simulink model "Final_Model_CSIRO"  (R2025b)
settings: Solver=ode23tb  StartTime=0.0  StopTime=50  RelTol=1e-3
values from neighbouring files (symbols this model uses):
  C_4 = 0.1670*C_b    (= 1.00487241952e-06)    [VSM_CSIRO.m]    (also in VSM.m)
  C_6 = 0.2835*C_b    (= 1.70587623314e-06)    [VSM_CSIRO.m]    (also in VSM.m)
  C_8 = 0.2275*C_b    (= 1.36891302659e-06)    [VSM_CSIRO.m]    (also in VSM.m)
  C_dc = 0.008*(n)    (= 1.6)    [VSM_CSIRO.m]    (also in VSM.m)
  C_f = n*300*10^-6    (= 0.06)    [VSM_CSIRO.m]    (also in VSM.m)
  D_p = (1/(m_p*w_b))    (= 101321.183642)    [VSM_CSIRO.m]    (also in VSM.m)
  droop_percentage = 1    [VSM_CSIRO.m]    (also in VSM.m = 5)
  i_ll = -1.15*(S_b/Vdc_n)-i_loss_dc    [VSM_CSIRO.m]    (also in VSM.m)
  i_ul = 1.15*(S_b/Vdc_n)+i_loss_dc    [VSM_CSIRO.m]    (also in VSM.m)
  J = D_p*tau_f    (= 2026.42367285)    [VSM_CSIRO.m]    (also in VSM.m)
  k_dc = eta_1/(Vdc_n*m_p)    [VSM_CSIRO.m]    (also in VSM.m)
  K_p = (1/Vdc_n)    [VSM_CSIRO.m]    (also in VSM.m)
  K_r = 1/R_dc    [VSM_CSIRO.m]    (also in VSM.m)
  Kff_i = 1    [VSM_CSIRO.m]    (also in VSM.m)
  Kff_v = 1    [VSM_CSIRO.m]    (also in VSM.m)
  Ki_i = (1/n)*1.19    (= 0.00595)    [VSM_CSIRO.m]    (also in VSM.m)
  Ki_v = (n)*1.161022    (= 232.2044)    [VSM_CSIRO.m]    (also in VSM.m)
  ki_v_ac = 4*5.2500e-04    (= 0.0021)    [VSM_CSIRO.m]    (also in VSM.m)
  Kp_i = 0.738891    [VSM_CSIRO.m]    (also in VSM.m)
  Kp_v = 0.52    [VSM_CSIRO.m]    (also in VSM.m)
  kp_v_ac = 0.001    [VSM_CSIRO.m]    (also in VSM.m)
  L1_pu = 1*0.0186/m    (= 0.000186)    [VSM_CSIRO.m]    (also in VSM.m)
  L_45 = L_lines(2)    [VSM_CSIRO.m]    (also in VSM.m)
  L_56 = L_lines(3)    [VSM_CSIRO.m]    (also in VSM.m)
  L_67 = L_lines(5)    [VSM_CSIRO.m]    (also in VSM.m)
  L_78 = L_lines(6)    [VSM_CSIRO.m]    (also in VSM.m)
  L_89 = L_lines(8)    [VSM_CSIRO.m]    (also in VSM.m)
  L_94 = L_lines(9)    [VSM_CSIRO.m]    (also in VSM.m)
  L_f = (1/n)*200*10^-6    (= 1e-06)    [VSM_CSIRO.m]    (also in VSM.m)
  n = 200    [VSM_CSIRO.m]    (also in VSM.m)
  pl = S_b*ps    (= 75000000)    [VSM_CSIRO.m]    (also in VSM.m)
  ps = base/3    (= 0.75)    [VSM_CSIRO.m]    (also in VSM.m)
  R1_pu = 1*0.00734/m    (= 7.34e-05)    [VSM_CSIRO.m]    (also in VSM.m)
  R_45 = R_lines(2)    [VSM_CSIRO.m]    (also in VSM.m)
  R_56 = R_lines(3)    [VSM_CSIRO.m]    (also in VSM.m)
  R_67 = R_lines(5)    [VSM_CSIRO.m]    (also in VSM.m)
  R_78 = R_lines(6)    [VSM_CSIRO.m]    (also in VSM.m)
  R_89 = R_lines(8)    [VSM_CSIRO.m]    (also in VSM.m)
  R_94 = R_lines(9)    [VSM_CSIRO.m]    (also in VSM.m)
  R_dc = (Vdc_n/(0.05*(S_b)/Vdc_n))    [VSM_CSIRO.m]    (also in VSM.m)
  R_f = 0.001/n    (= 5e-06)    [VSM_CSIRO.m]    (also in VSM.m)
  S_b = 100*(10^6)    (= 100000000)    [VSM_CSIRO.m]    (also in VSM.m)
  S_bt = S_b    (= 100000000)    [VSM_CSIRO.m]    (also in VSM.m)
  T_en = T_load-0.5    (= 44.5)    [VSM_CSIRO.m]    (also in VSM.m = 24.5)
  t_l = 2    [VSM_CSIRO.m]
  tau_dc = 0.05    [VSM_CSIRO.m]    (also in VSM.m)
  tau_g = 5    [VSM_CSIRO.m]    (also in VSM.m)
  V1_rms = 1000    [VSM_CSIRO.m]    (also in VSM.m)
  V2_rms = 13800    [VSM_CSIRO.m]    (also in VSM.m)
  V_m = sqrt(2/3)*V1_rms    [VSM_CSIRO.m]    (also in VSM.m)
  Vdc_n = 3*V_m    [VSM_CSIRO.m]    (also in VSM.m)
  w_b = 2*pi*f_b    (= 314.159265359)    [VSM_CSIRO.m]    (also in VSM.m)
  w_f = 2*pi*5    (= 31.4159265359)    [VSM_CSIRO.m]    (also in VSM.m)
undefined symbols (not defined in the file or in its folder): D1, Delta, DiscIntNeverNeededParam, i_dc
libraries: spsSeriesRLCBranchLib x142, spsThreePhaseVIMeasurementLib x69, slpidlib x44, spsabctodq0Lib x44, spsVoltageMeasurementLib x28, spsGroundLib x23, spsThreePhaseBreakerLib x23, spsThreePhaseParallelRLCLoadLib x21, spsdq0toabcLib x16, spsUniversalBridgeLib x16, spsPowerPositiveSequenceLib x14, spsDCVoltageSourceLib x14
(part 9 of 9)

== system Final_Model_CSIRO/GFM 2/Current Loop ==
  i_s_ref_dq0 : Inport
  v_dq0 : Inport  Port=2
  i_s_dq0 : Inport  Port=3
  w : Inport  Port=4
  Demux : Demux  Outputs=2
  Demux1 : Demux  Outputs=2
  Demux2 : Demux  Outputs=2
  First-Order Filter2 : spsFirstOrderFilterLib/First-Order Filter  Commented=on  FilterType=Lowpass  Tc=25e-3  Ts=0  Initialize=on  Vac_Init=[0, 0, 50]  Vdc_Init=1  PlotResponse=off  FreqRange="[0,  200,  1]"
  First-Order Filter3 : spsFirstOrderFilterLib/First-Order Filter  Commented=on  FilterType=Lowpass  Tc=25e-3  Ts=0  Initialize=on  Vac_Init=[0, 0, 50]  Vdc_Init=0  PlotResponse=off  FreqRange="[0,  200,  1]"
  Gain Corrector : Gain  Gain=Kp_i
  Gain Corrector1 : Gain  Gain=Kp_i
  Integration Time : Gain  Gain=Ki_i / Kp_i
  Integration Time 1 : Gain  Gain=Ki_i / Kp_i
  Integration Time1 : Gain  Gain=1/n
  Integration Time2 : Gain  Gain=1/n
  Integrator : Integrator  InitialCondition=0.0001
  Integrator 1 : Integrator
  Mux : Mux  Inputs=3
  Product : Product  RndMeth=Zero
  Product1 : Product  RndMeth=Zero
  Selector1 : Selector  InputPortWidth=3  IndexOptions=Index vector (dialog)  Indices=[1 2]  OutputSizes=1
  Selector2 : Selector  InputPortWidth=3  IndexOptions=Index vector (dialog)  Indices=[1 2]  OutputSizes=1
  Selector3 : Selector  InputPortWidth=3  IndexOptions=Index vector (dialog)  Indices=[1 2]  OutputSizes=1
  Sum : Sum  Inputs=|+-
  Sum1 : Sum  Inputs=|++
  Sum2 : Sum  Inputs=|+-
  Sum3 : Sum  Inputs=|++
  Sum4 : Sum  Inputs=|++
  Sum5 : Sum  Inputs=++|
  Sum6 : Sum  Inputs=-+|
  Sum7 : Sum  Inputs=++|
  Vm_0* : Constant  Value=0
  Voltage Compensator 1 : Gain  Gain=Kff_v
  Voltage compensator : Gain  Gain=Kff_v
  w*Lf_pu : Gain  Gain=L_f
  v_s_ref_dq0 : Outport  VectorParamsAs1DForOutWhenUnconnected=off
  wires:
  Integration Time2/1 -> Sum4/2
  Integration Time1/1 -> Sum1/2
  Gain Corrector1/1 -> Sum5/2
  Product1/1 -> Sum5/1
  Demux2/1 -> Voltage compensator/1
  Demux1/1 -> Sum/2, Product1/2
  Integrator/1 -> Sum1/1
  Vm_0*/1 -> Mux/3
  Demux1/2 -> Sum6/1, Product/1
  Selector3/1 -> Demux2/1
  i_s_dq0/1 -> Selector2/1
  Selector2/1 -> Demux1/1
  Mux/1 -> v_s_ref_dq0/1
  w/1 -> w*Lf_pu/1
  Gain Corrector/1 -> Sum2/1
  Selector1/1 -> Demux/1
  Demux/2 -> Sum6/2
  Sum4/1 -> Gain Corrector1/1
  Sum2/1 -> Sum3/1
  Sum1/1 -> Gain Corrector/1
  Voltage compensator/1 -> Sum3/2
  Integrator 1/1 -> Sum4/1
  v_dq0/1 -> Selector3/1
  i_s_ref_dq0/1 -> Selector1/1
  w*Lf_pu/1 -> Product/2, Product1/1
  Product/1 -> Sum2/2
  Voltage Compensator 1/1 -> Sum7/1
  Demux2/2 -> Voltage Compensator 1/1
  Sum7/1 -> Mux/2  "Vm_q*"
  Sum3/1 -> Mux/1  "Vm_d*"
  Demux/1 -> Sum/1
  Sum6/1 -> Integration Time2/1, Integration Time 1/1
  Sum5/1 -> Sum7/2
  Integration Time/1 -> Integrator/1
  Integration Time 1/1 -> Integrator 1/1
  Sum/1 -> Integration Time1/1, Integration Time/1

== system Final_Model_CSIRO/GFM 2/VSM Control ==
  p_m : Inport
  p_set : Inport  Port=2
  v_m : Inport  Port=3
  V_abc : Inport  Port=4
  w_b : Inport  Port=5
  Demux : Demux  Outputs=3
  Gain17 : Gain  Gain=1/(w_b)
  Gain2 : Gain  Gain=1/(w_b)
  Gain5 : Gain  Gain=D_p
  Gain6 : Gain  Gain=1/J
  Integrator : Integrator
  Integrator2 : Integrator
  MATLAB Function1 : MATLAB Function  TreatAsAtomicUnit=on
  PID Controller : slpidlib/PID Controller  Controller=PID  Form=Parallel  TimeDomain=Continuous-time  UseExternalTs=off  SampleTime=-1  IntegratorMethod=Forward Euler  FilterMethod=Forward Euler  ControllerParametersSource=internal  P=kp_v_ac  I=ki_v_ac  UseKiTs=off  D=0  UseExternalDerivativeSource=off  N=100  UseFilter=on  TunerSelectOption=Transfer Function Based (PID Tuner App)  InitialConditionSource=internal  InitialConditionForIntegrator=0  InitialConditionForFilter=0  DifferentiatorICPrevScaledInput=0  ExternalReset=none  TrackingMode=off  Kt=1  LimitOutput=off  SatLimitsSource=internal  UpperSaturationLimit=inf  LowerSaturationLimit=-inf  LinearizeAsGain=on  AntiWindupMode=none  Kb=1  LimitIntegrator=off  UpperIntegratorSaturationLimit=inf  LowerIntegratorSaturationLimit=-inf  POutMin=[]  POutMax=[]  IOutMin=[]  IOutMax=[]  DOutMin=[]  DOutMax=[]  NOutMin=[]  NOutMax=[]  SumOutMin=[]  SumOutMax=[]  SaturationOutMin=[]  SaturationOutMax=[]  PParamMin=[]  PParamMax=[]  IParamMin=[]  IParamMax=[]  DParamMin=[]  DParamMax=[]  NParamMin=[]  NParamMax=[]  KbParamMin=[]  KbParamMax=[]  KtParamMin=[]  KtParamMax=[]  KbOutMin=[]  KbOutMax=[]  KtOutMin=[]  KtOutMax=[]  IntegratorOutMin=[]  IntegratorOutMax=[]  FilterOutMin=[]  FilterOutMax=[]  SumI1OutMin=[]  SumI1OutMax=[]  SumI2OutMin=[]  SumI2OutMax=[]  SumI3OutMin=[]  SumI3OutMax=[]  SumI4OutMin=[]  SumI4OutMax=[]  SumDOutMin=[]  SumDOutMax=[]  DifferentiatorOutMin=[]  DifferentiatorOutMax=[]  FilterDiffOutCoefMin=[]  FilterDiffOutCoefMax=[]  ReciprocalOutMin=[]  ReciprocalOutMax=[]  SumDenOutMin=[]  SumDenOutMax=[]  SumNumOutMin=[]  SumNumOutMax=[]  DivideOutMin=[]  DivideOutMax=[]  UdiffTsProdOutMin=[]  UdiffTsProdOutMax=[]  NTsProdOutMin=[]  NTsProdOutMax=[]  UintegralTsProdOutMin=[]  UintegralTsProdOutMax=[]  UngainTsProdOutMin=[]  UngainTsProdOutMax=[]  ClampingZeroOutDataTypeStr=Inherit: Inherit via back propagation  ClampingZeroOutMin=[]  ClampingZeroOutMax=[]  FilterDenConstantOutDataTypeStr=Inherit: Inherit via back propagation  FilterDenConstantOutMin=[]  FilterDenConstantOutMax=[]  PCopyOutDataTypeStr=Inherit: Inherit via back propagation  PCopyOutMin=[]  PCopyOutMax=[]  NCopyOutDataTypeStr=Inherit: Inherit via back propagation  NCopyOutMin=[]  NCopyOutMax=[]  IntegratorContinuousStateAttributes=''  IntegratorStateMustResolveToSignalObject=off  IntegratorRTWStateStorageClass=Auto  FilterContinuousStateAttributes=''  FilterStateMustResolveToSignalObject=off  FilterRTWStateStorageClass=Auto  ParallelPVariant=InternalParameters  IdealPVariant=Disabled  IVariant=InternalParameters  DVariant=InternalParameters  IntegratorVariant=Continuous  SatVariant=Disabled  AWVariant=Passthrough  PCopyVariant=Disabled  TRVariant=Disabled  FdbkBlocksVariant=Forward  IdealPFdbkVariant=Disabled  SatFdbkVariant=Disabled  DerivativeFilterVariant=ContFilter  NVariant=InternalParameters  NCopyVariant=Disabled  FilterICVariant=InternalICsFilter  IntegratorICVariant=InternalICs  ExternalResetVariant=Disabled  TRSumVariant=Passthrough  SumFdbkVariant=Disabled  SumVariant=Sum_PID  TsampFilterVariant=InternalTs  TsampNgainVariant=Passthrough  TsampIntegralVariant=Disabled_SignalSpec  ExternalSaturationOutDataTypeStr=Inherit: Same as second input  DerivativeSourceVariant=ErrorSignal  PreIntVariant=InternalPreInt
  Sum : Sum  Inputs=+|+|-
  Sum1 : Sum  Inputs=-+|
  Sum2 : Sum  Inputs=+|-
  Terminator : Terminator
  Terminator1 : Terminator
  Transfer Fcn1 : TransferFcn  Numerator=[w_f]  Denominator=[1 w_f]
  abc to dq1 : spsabctodq0Lib/abc to dq0  Alignment=90 degrees behind phase A axis
  abc to dq2 : spsabctodq0Lib/abc to dq0  Alignment=90 degrees behind phase A axis
  w_ref : Outport  VectorParamsAs1DForOutWhenUnconnected=off
  theta_ref : Outport  Port=2  VectorParamsAs1DForOutWhenUnconnected=off
  v_ref_dq0 : Outport  Port=3  VectorParamsAs1DForOutWhenUnconnected=off
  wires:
  v_m/1 -> Sum1/2
  Sum1/1 -> PID Controller/1
  abc to dq1/1 -> Demux/1
  V_abc/1 -> abc to dq1/1
  Demux/1 -> Sum1/1
  Demux/2 -> Terminator/1
  Demux/3 -> Terminator1/1
  w_b/1 -> Sum2/1
  Integrator/1 -> Integrator2/1, Sum2/2, w_ref/1, MATLAB Function1/3(w)
  Transfer Fcn1/1 -> Gain17/1
  Integrator2/1 -> abc to dq1/2, MATLAB Function1/2(theta), abc to dq2/2, theta_ref/1
  Sum2/1 -> Gain5/1
  Sum/1 -> Gain6/1
  Gain2/1 -> Sum/2
  Gain6/1 -> Integrator/1
  Gain17/1 -> Sum/3
  Gain5/1 -> Sum/1
  p_m/1 -> Transfer Fcn1/1
  p_set/1 -> Gain2/1
  PID Controller/1 -> MATLAB Function1/1(M_fi_f)
  MATLAB Function1/1(e) -> abc to dq2/1
  abc to dq2/1 -> v_ref_dq0/1

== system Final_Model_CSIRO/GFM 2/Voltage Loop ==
  v_ref_dq0 : Inport
  v_dq0 : Inport  Port=2
  i_dq0 : Inport  Port=3
  w : Inport  Port=4
  Current Compensator : Gain  Gain=Kff_i
  Current Compensator1 : Gain  Gain=Kff_i
  Damping (d) : Gain  Gain=Kp_v
  Damping (q) : Gain  Gain=Kp_v
  Demux : Demux  Outputs=2
  Demux1 : Demux  Outputs=2
  Demux2 : Demux  Outputs=2
  Eg_d * (wCf) : Product  RndMeth=Zero
  "Eg_q * (wCf) " : Product  RndMeth=Zero
  Filter capacitance : Gain  Gain=C_f
  Integration Time : Gain  Gain=Ki_v / Kp_v
  Integration Time1 : Gain  Gain=Ki_v / Kp_v
  Integration Time2 : Gain  Gain=n
  Integration Time3 : Gain  Gain=n
  Integrator : Integrator
  Integrator1 : Integrator
  Is_0* : Constant  Value=0
  Mux : Mux  Inputs=3
  Selector : Selector  InputPortWidth=3  IndexOptions=Index vector (dialog)  Indices=[1 2]  OutputSizes=1
  Selector1 : Selector  InputPortWidth=3  IndexOptions=Index vector (dialog)  Indices=[1 2]  OutputSizes=1
  Selector2 : Selector  InputPortWidth=3  IndexOptions=Index vector (dialog)  Indices=[1 2]  OutputSizes=1
  Sum : Sum  Inputs=|+-
  Sum1 : Sum  Inputs=|++
  Sum2 : Sum  Inputs=|+-
  Sum3 : Sum  Inputs=|++
  Sum4 : Sum  Inputs=|++
  Sum5 : Sum  Inputs=++|
  Sum6 : Sum  Inputs=-+|
  Sum7 : Sum  Inputs=++|
  i_s_ref_dq0 : Outport  VectorParamsAs1DForOutWhenUnconnected=off
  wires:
  Integration Time3/1 -> Sum4/2
  Integration Time2/1 -> Sum1/2
  Sum/1 -> Integration Time2/1, Integration Time/1
  Mux/1 -> i_s_ref_dq0/1
  Selector2/1 -> Demux2/1
  Selector1/1 -> Demux/1
  Selector/1 -> Demux1/1
  Damping (q)/1 -> Sum5/2  "Is_q\""
  v_dq0/1 -> Selector/1
  Sum3/1 -> Mux/1  "Is_d*"
  Sum4/1 -> Damping (q)/1
  Integration Time/1 -> Integrator/1
  Integrator/1 -> Sum1/1
  Sum1/1 -> Damping (d)/1
  Sum5/1 -> Sum7/2  "Is_q'"
  i_dq0/1 -> Selector2/1
  Damping (d)/1 -> Sum2/1  "Is_d\""
  Filter capacitance/1 -> Eg_d * (wCf)/2, "Eg_q * (wCf) "/2
  Demux1/2 -> Sum6/1, "Eg_q * (wCf) "/1  "Eg_q"
  "Eg_q * (wCf) "/1 -> Sum2/2  "Is_f"
  Current Compensator1/1 -> Sum7/1
  Demux1/1 -> Sum/2, Eg_d * (wCf)/1  "Eg_d"
  Current Compensator/1 -> Sum3/2
  Sum2/1 -> Sum3/1  "Is_d'"
  Demux2/1 -> Current Compensator/1  "Ig_d"
  Sum6/1 -> Integration Time1/1, Integration Time3/1
  Demux/1 -> Sum/1  "Eg_d*"
  Demux2/2 -> Current Compensator1/1  "Ig_q"
  Sum7/1 -> Mux/2  "Is_q*"
  Eg_d * (wCf)/1 -> Sum5/1  "Is_f"
  v_ref_dq0/1 -> Selector1/1
  Demux/2 -> Sum6/2  "Eg_q*"
  Integrator1/1 -> Sum4/1
  Integration Time1/1 -> Integrator1/1
  w/1 -> Filter capacitance/1
  Is_0*/1 -> Mux/3

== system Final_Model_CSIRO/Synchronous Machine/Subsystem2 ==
  P_ref : Inport
  speed_ref : Inport  Port=2
  speed : Inport  Port=3
  1/droop : Gain  Gain=1/((droop_percentage/100))
  Delta load setpoint : Sum  Inputs=+-|
  Delta speed : Sum  Inputs=-+|
  throttle : Outport  VectorParamsAs1DForOutWhenUnconnected=off
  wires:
  speed/1 -> Delta speed/2
  1/droop/1 -> Delta load setpoint/2
  Delta speed/1 -> 1/droop/1
  speed_ref/1 -> Delta speed/1
  P_ref/1 -> Delta load setpoint/1
  Delta load setpoint/1 -> throttle/1

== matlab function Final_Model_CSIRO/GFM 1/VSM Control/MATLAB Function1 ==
function e = EMF(M_fi_f,theta,w)
e=w*M_fi_f*[sin(theta) sin(theta-(2*pi/3)) sin(theta-(4*pi/3))]';
end

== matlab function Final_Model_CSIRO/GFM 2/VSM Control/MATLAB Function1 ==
function e = EMF(M_fi_f,theta,w)
e=w*M_fi_f*[sin(theta) sin(theta-(2*pi/3)) sin(theta-(4*pi/3))]';
end

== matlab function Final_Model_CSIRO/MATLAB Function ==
function [SCR, Ipeak, Isc, Ssc] = fcn(Ia, Ib, Ic)
% MATLAB Function block version that holds the peak over simulation

% persistent variable to store max current
persistent Ipeak_prev

% Initialize at the first step
if isempty(Ipeak_prev)
    Ipeak_prev = 0;
end

% Current sample magnitude
Icurr = max([abs(Ia), abs(Ib), abs(Ic)]); % assumes scalar input per time step

% Update peak if current > previous
Ipeak_prev = max(Ipeak_prev, Icurr);

% Output current peak
Ipeak = Ipeak_prev;

% Convert to RMS
Isc = Ipeak / sqrt(2);

% Rated line-line voltage
Vll = 13.8e3;     % volts

% Inverters rated power
S_rated = (10e6)+(110e6); % VA

% Short-circuit apparent power
Ssc = sqrt(3)*Vll*Isc;

% SCR
SCR = Ssc / S_rated;
